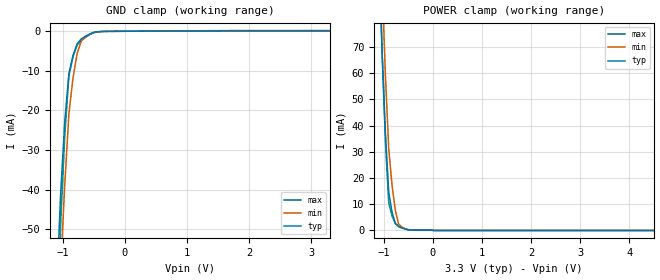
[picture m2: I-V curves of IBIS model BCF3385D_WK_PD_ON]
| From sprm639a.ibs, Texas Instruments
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|   Model Cell BCF3385D_WK_PD_ON
|BCF3385D_WK_PD_ON
[Model]   BCF3385D_WK_PD_ON
Model_type   Input
Polarity   Non-Inverting
Vinl =  0.8
Vinh =  2
C_comp   1.187844p   1.059102p   1.312744p
[Model Spec]
Vinl   0.8   0.8   0.8
Vinh   2   2   2
[Temperature Range]   25   155   -40
[Voltage Range]   3.3   2.97   3.63
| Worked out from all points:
|   GND clamp passes 1 mA (typ) near -0.60 V on its own axis
|   POWER clamp passes 1 mA (typ) near -0.64 V on its own axis
| Nom Voltages:
|   VDD=1.2, VDDS=3.3, VSS=0
| Min Voltages:
|   VDD=1.08, VDDS=2.97, VSS=0
| Max Voltages:
|   VDD=1.32, VDDS=3.63, VSS=0
[POWER_clamp]
|   voltage   I(typ)   I(min)   I(max)
-3.3V     1.862A     2.383A     2.005A
-1.1V     105.6mA    134.9mA    109.7mA
-1.033V   67.09mA    93.26mA    66.5mA
-966.7mV  36.71mA    58.64mA    33.42mA
-900mV    14.43mA    31.04mA    10.5mA
-833.3mV  7.051mA    17.26mA    5.544mA
-766.7mV  2.715mA    7.751mA    2.645mA
-700mV    1.423mA    2.498mA    1.797mA
-566.7mV  522.6uA    583.3uA    687.1uA
-366.7mV  113.8uA    74.21uA    183.7uA
6.6V      0A         0A         0A
[GND_clamp]
|   voltage   I(typ)   I(min)   I(max)
-3.3V     -1.421A    -1.358A    -2.122A
-1.1V     -65.92mA   -84.59mA   -78.36mA
-1.033V   -41.09mA   -60mA      -48.66mA
-966.7mV  -22.68mA   -38.72mA   -26.26mA
-900mV    -10.68mA   -20.73mA   -11.17mA
-833.3mV  -6.049mA   -11.65mA   -6.382mA
-766.7mV  -3.124mA   -5.534mA   -3.441mA
-700mV    -1.909mA   -2.394mA   -2.347mA
-566.7mV  -705.7uA   -768.6uA   -867.7uA
-500mV    -273.5uA   -349.1uA   -323.9uA
-300mV    -27.98uA   -20.36uA   -40.75uA
3.3V      107.2uA    57.97uA    177.9uA
